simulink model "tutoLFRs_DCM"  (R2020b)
settings: Solver=VariableStepAuto  StartTime=0.0  StopTime=10.0  RelTol=1e-3
undefined symbols (not defined in the file): sig2
libraries: RCTblocks x2

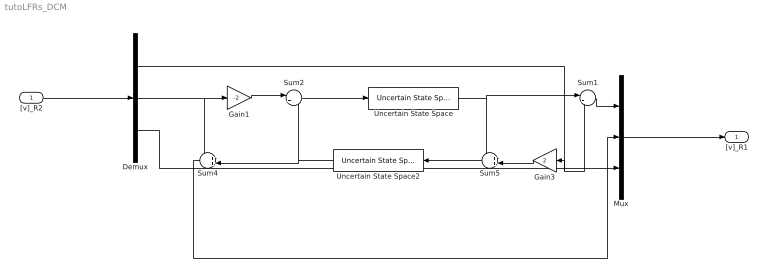
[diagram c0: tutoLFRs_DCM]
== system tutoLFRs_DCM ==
  "[v]_R2" : Inport  OutDataTypeStr=double  PortDimensions=3
  Demux : Demux  Outputs=3
  Gain1 : Gain  Gain=-2
  Gain3 : Gain  Gain=2
  Mux : Mux  Inputs=3
  Sum1 : Sum  Inputs=|++
  Sum2 : Sum  Inputs=|+-
  Sum4 : Sum  Inputs=++|
  Sum5 : Sum  Inputs=++|
  Uncertain State Space : RCTblocks/Uncertain State Space  Tag=USS  USystem=ss(sig2)  UValue=[]  X0=[]  uX0=[]
  Uncertain State Space2 : RCTblocks/Uncertain State Space  Tag=USS  USystem=ss(sig2)  UValue=[]  X0=[]  uX0=[]
  "[v]_R1" : Outport  VectorParamsAs1DForOutWhenUnconnected=off
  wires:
  Sum1/1 -> Mux/1
  Gain3/1 -> Sum5/2
  Demux/2 -> Sum4/1, Gain1/1
  Sum2/1 -> Uncertain State Space/1
  Demux/1 -> Gain3/1, Sum1/2
  Gain1/1 -> Sum2/1
  Demux/3 -> Mux/3
  Sum5/1 -> Uncertain State Space2/1
  Uncertain State Space2/1 -> Sum4/2, Sum2/2
  Sum4/1 -> Mux/2
  Mux/1 -> "[v]_R1"/1
  Uncertain State Space/1 -> Sum5/1, Sum1/1
  "[v]_R2"/1 -> Demux/1
